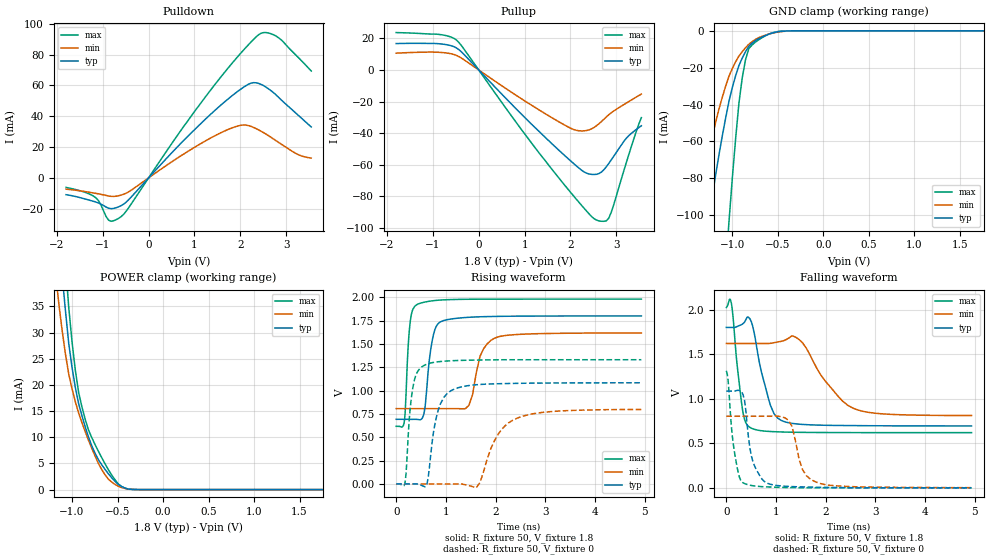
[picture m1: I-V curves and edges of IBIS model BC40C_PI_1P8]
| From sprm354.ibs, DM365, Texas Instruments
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|NO_TERM_SSTL_0.1_1P5
|BUFFER OPERATING UNDER NO TERMINATION MODE AND SSTL RECIVER MODE WITH
| 1.5V SUPPLY WITH +/-0.1V VARIATION
|   Model Cell BC40C_PI_1P8
|BC1833DV40CTHYPBFZP_PI_1P8
[Model]   BC40C_PI_1P8
Model_type   I/O
Polarity   Non-Inverting
Enable   Active-Low
Vinl =  0.63V
Vinh =  1.17V
Cref =  15pF
Rref =  100.00M
Vref =  0V
Vmeas =  0.9
C_comp   2.12243p   1.981083p   2.174981p
[Model Spec]
Vinl   0.63V   0.567V   0.693V
Vinh   1.17V   1.053V   1.287V
[Temperature Range]   25   125   -40
[Voltage Range]   1.8   1.62   1.98
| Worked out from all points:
|   slope of the pulldown table from 0 to 0.27 V, typ, clamps not added: 30.7 ohm
|   slope of the pullup table from 0 to 0.27 V, typ, clamps not added: 32.7 ohm
|   GND clamp passes 1 mA (typ) near -0.54 V on its own axis
|   POWER clamp passes 1 mA (typ) near -0.49 V on its own axis
|   rising waveform, R_fixture 50, V_fixture 1.8: 20-80 % time 144ps typ, 227ps min, 84.7ps max; typ from 0.692 V to 1.8 V
|   rising waveform, R_fixture 50, V_fixture 0: 20-80 % time 223ps typ, 452ps min, 131ps max; typ from 0 V to 1.08 V
|   falling waveform, R_fixture 50, V_fixture 1.8: 20-80 % time 284ps typ, 626ps min, 159ps max; typ from 1.8 V to 0.695 V
|   falling waveform, R_fixture 50, V_fixture 0: 20-80 % time 201ps typ, 240ps min, 150ps max; typ from 1.08 V to 0 V
[POWER_clamp]
|   voltage   I(typ)   I(min)   I(max)
-1.8V     222.8mA    182.4mA    260.3mA
-1.182V   57.15mA    41.74mA    71.93mA
-1.145V   48.76mA    35.58mA    61.82mA
-1.109V   41.19mA    30.47mA    52.31mA
-1.073V   34.25mA    25.98mA    43.33mA
-1.036V   27.96mA    22.09mA    34.87mA
-963.6mV  19.52mA    16.79mA    22.82mA
-854.5mV  11.96mA    11.06mA    13.39mA
-709.1mV  5.681mA    4.97mA     7.285mA
-527.3mV  1.582mA    996.7uA    1.871mA
-345.5mV  54.71uA    54.7uA     36.19uA
1.764V    -856.8pA   -880.6nA   -264.9pA
[Pulldown]
|   voltage   I(typ)   I(min)   I(max)
-1.8V     -10.95mA   -7.357mA   -6.223mA
-1.145V   -15.77mA   -10.12mA   -13.08mA
-872.7mV  -19.73mA   -11.78mA   -27.47mA
-600mV    -18.04mA   -11.2mA    -25.16mA
763.6mV   24.27mA    15.41mA    33.34mA
1.636V    48.77mA    30.11mA    67.73mA
1.964V    56.56mA    33.79mA    79.35mA
2.182V    60.82mA    33.86mA    86.53mA
2.455V    60.6mA     30.18mA    93.85mA
2.836V    52.14mA    22.94mA    90.8mA
3.273V    40.32mA    14.9mA     77.8mA
3.545V    32.99mA    12.81mA    69.32mA
[Pullup]
|   voltage   I(typ)   I(min)   I(max)
-1.8V     16.74mA    10.66mA    23.69mA
-872.7mV  16.63mA    11.2mA     22.53mA
-490.9mV  14.03mA    9.282mA    19.05mA
981.8mV   -29.42mA   -19.17mA   -39.71mA
1.964V    -56.5mA    -36.27mA   -76.09mA
2.291V    -64.43mA   -38.53mA   -87.31mA
2.564V    -66.04mA   -35.36mA   -94.96mA
2.727V    -63.17mA   -31.2mA    -95.76mA
2.836V    -59.06mA   -28.31mA   -93.71mA
2.945V    -54.5mA    -25.9mA    -85.05mA
3.218V    -43.17mA   -20.92mA   -58.52mA
3.545V    -35.29mA   -15.24mA   -30.18mA
[GND_clamp]
|   voltage   I(typ)   I(min)   I(max)
-1.8V     -283.9mA   -196.9mA   -714.1mA
-1.436V   -160mA     -106.5mA   -417.6mA
-1.291V   -112.1mA   -72.7mA    -299.5mA
-1.255V   -100.4mA   -64.61mA   -270.2mA
-1.036V   -38.24mA   -24.67mA   -103.6mA
-963.6mV  -24.43mA   -16.85mA   -58.82mA
-927.3mV  -18.91mA   -13.72mA   -39.41mA
-890.9mV  -14.81mA   -11.33mA   -25.62mA
-818.2mV  -8.414mA   -7.299mA   -9.624mA
-745.5mV  -5.28mA    -4.675mA   -6.094mA
-454.5mV  -257uA     -378.6uA   -188.6uA
1.764V    13.55nA    514.3nA    10.43nA
[Ramp]
| variable   typ   min   max
dV/dt_f  0.7341562/0.297695n   0.5392068/0.6628642n  0.8999709/0.164724n
dV/dt_r  0.6697522/0.2220131n  0.5074972/0.459599n   0.8112485/0.1302976n
R_load = 50
[Rising Waveform]
R_fixture = 50
V_fixture = 1.8
V_fixture_min = 1.62
V_fixture_max = 1.98
|   time   V(typ)   V(min)   V(max)
0s        692.3mV    806.8mV    617mV
156ps     692.3mV    806.8mV    645.5mV
282ps     691.9mV    806.8mV    1.738V
420ps     691.6mV    806.8mV    1.922V
558ps     750.8mV    806.8mV    1.946V
720ps     1.523V     806.8mV    1.961V
888ps     1.736V     806.8mV    1.97V
1.464ns   1.785V     843.5mV    1.979V
2.046ns   1.795V     1.575V     1.98V
4.932ns   1.8V       1.617V     1.98V
[Rising Waveform]
R_fixture = 50
V_fixture = 0
V_fixture_min = 0
V_fixture_max = 0
|   time   V(typ)   V(min)   V(max)
0s        14.78uV    -341.1nV   -541.5uV
168ps     9.981uV    9.295uV    -6.905mV
336ps     -445.9uV   10.17uV    1.035V
582ps     -30.81mV   9.894uV    1.275V
834ps     768.8mV    11.63uV    1.308V
1.104ns   999.6mV    -311.7uV   1.319V
1.608ns   1.062V     -42.31mV   1.327V
2.046ns   1.073V     528.3mV    1.33V
2.442ns   1.078V     706.7mV    1.33V
4.932ns   1.083V     797mV      1.331V
[Falling Waveform]
R_fixture = 50
V_fixture = 1.8
V_fixture_min = 1.62
V_fixture_max = 1.98
|   time   V(typ)   V(min)   V(max)
0s        1.8V       1.62V      2.023V
102ps     1.8V       1.62V      2.07V
324ps     1.837V     1.62V      883.3mV
504ps     1.862V     1.62V      669.4mV
888ps     925.1mV    1.621V     632.3mV
1.104ns   756.7mV    1.644V     627.2mV
1.464ns   714.6mV    1.664V     623mV
1.974ns   702.3mV    1.21V      620.9mV
2.55ns    698.8mV    893.6mV    620mV
4.932ns   694.8mV    811.9mV    619.4mV
[Falling Waveform]
R_fixture = 50
V_fixture = 0
V_fixture_min = 0
V_fixture_max = 0
|   time   V(typ)   V(min)   V(max)
0s        1.085V     803.5mV    1.314V
168ps     1.085V     803.4mV    386.2mV
264ps     1.092V     803.4mV    119.2mV
366ps     982.2mV    803.5mV    48.51mV
528ps     307.6mV    803.5mV    24.33mV
834ps     49.95mV    803.4mV    10.38mV
1.248ns   16.2mV     759.4mV    3.492mV
1.536ns   10.38mV    202.3mV    1.51mV
1.83ns    6.976mV    59.94mV    635.9uV
4.932ns   282.7uV    2.919mV    5.957uV
